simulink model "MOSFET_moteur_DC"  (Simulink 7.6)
settings: Solver=ode15s  StartTime=0.0  StopTime=0.1  RelTol=1e-3
InitFcn:
  | clc, close all
StopFcn:
  | close all, clc
  | load signaux_VitPos.mat
  | plotyy(x(1,:),x(2,:),x(1,:),x(3,:))
  | grid
  | title('Vitesse (rad/s) et Angle de rotation (rad)')
  | 
  | figure
  | load signaux_VI.mat
  | subplot 212
  | plot(y(1,:),y(2,:))
  | title('Courant de drain Id (A)')
  | grid
  | subplot 211
  | plot (y(1,:),y(3,:))
  | grid
  | title('Tension PWM de grille (V)')
libraries: fl_lib x14, nesl_utility x6, elec_lib x5

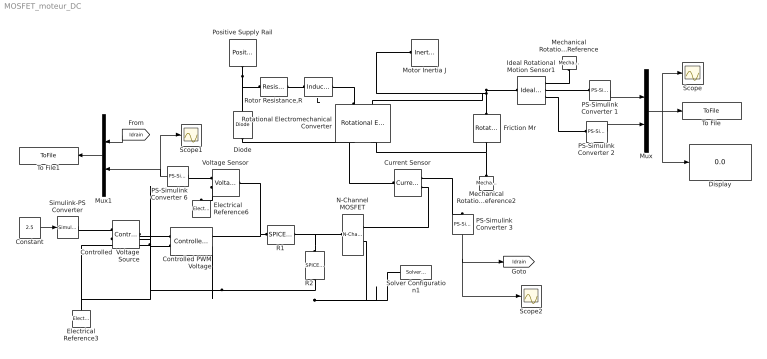
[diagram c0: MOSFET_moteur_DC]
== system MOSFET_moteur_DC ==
  Constant : Constant  Value=2.5
  Controlled  Voltage Source : fl_lib/Electrical/Electrical Sources/Controlled Voltage Source  DialogController=NetworkEngine.DynNeDlgSource  SystemSampleTime=-1  i_Log=off  v_Log=off  LocalVarNames=|i|v  LocalVarDescs=|i|v  LocalVarLogging=[0 0]
  Controlled PWM Voltage : elec_lib/Actuators & Drivers/Drivers/Controlled PWM Voltage  DialogController=NetworkEngine.DynNeDlgSource  SystemSampleTime=-1  F=1000 Hz  Vmin=0 V  Vmax=5 V  Vm=5 V  pwm_or_av=1  current_Log=off  voltage_Log=off  power_Log=off  LocalVarNames=|current|voltage|power  LocalVarDescs=|Load current (A)|Load voltage (V)|Load power (W)  LocalVarLogging=[0 0 0]
  Current Sensor : fl_lib/Electrical/Electrical Sensors/Current Sensor  DialogController=NetworkEngine.DynNeDlgSource  SystemSampleTime=-1  i1_Log=off  v1_Log=off  LocalVarNames=|i1|v1  LocalVarDescs=|i1|v1  LocalVarLogging=[0 0]
  Diode : fl_lib/Electrical/Electrical Elements/Diode  DialogController=NetworkEngine.DynNeDlgSource  SystemSampleTime=-1  Vf=0.6 V  Ron=0.3 Ohm  Goff=1e-08 1/Ohm  i_Log=off  v_Log=off  LocalVarNames=|i|v  LocalVarDescs=|i|v  LocalVarLogging=[0 0]
  Display : Display
  Electrical Reference3 : fl_lib/Electrical/Electrical Elements/Electrical Reference  DialogController=NetworkEngine.DynNeDlgSource  SystemSampleTime=-1  i_Log=off  LocalVarNames=|i  LocalVarDescs=|i  LocalVarLogging=[]
  Electrical Reference6 : fl_lib/Electrical/Electrical Elements/Electrical Reference  DialogController=NetworkEngine.DynNeDlgSource  SystemSampleTime=-1  i_Log=off  LocalVarNames=|i  LocalVarDescs=|i  LocalVarLogging=[]
  Friction Mr : fl_lib/Mechanical/Rotational Elements/Rotational Friction  DialogController=NetworkEngine.DynNeDlgSource  SystemSampleTime=-1  brkwy_trq=0.02e-3 N*m  Col_trq=0.02e-3 N*m  visc_coef=0 N*m/(rad/s)  trans_coef=10 s/rad  vel_thr=0.1 rad/s  t_Log=off  w_Log=off  LocalVarNames=|friction_torque|rel_velocity|power  LocalVarDescs=|Friction torque (N*m)|Relative velocity (rad/s)|Power (W)  LocalVarLogging=[0 0 0]
  Ideal Rotational Motion Sensor1 : fl_lib/Mechanical/Mechanical Sensors/Ideal Rotational Motion Sensor  DialogController=NetworkEngine.DynNeDlgSource  SystemSampleTime=-1  offset=0 rad  w_Log=off  t_Log=off  phi_Log=off  LocalVarNames=|w|t|phi  LocalVarDescs=|w|t|phi  LocalVarLogging=[]
  L : fl_lib/Electrical/Electrical Elements/Inductor  DialogController=NetworkEngine.DynNeDlgSource  SystemSampleTime=-1  l=12e-6 H  i0=0 A  r=0 Ohm  g=1e-09 1/Ohm  i_Log=off  v_Log=off  i_L_Log=off  LocalVarNames=|current|voltage|power  LocalVarDescs=|Inductor current (A) |Voltage across inductor (V)|Power (W)  LocalVarLogging=[0 0 0]
  Mechanical Rotational Reference : fl_lib/Mechanical/Rotational Elements/Mechanical Rotational Reference  DialogController=NetworkEngine.DynNeDlgSource  SystemSampleTime=-1  t_Log=off  LocalVarNames=|t  LocalVarDescs=|t  LocalVarLogging=[]
  Mechanical Rotational Reference2 : fl_lib/Mechanical/Rotational Elements/Mechanical Rotational Reference  DialogController=NetworkEngine.DynNeDlgSource  SystemSampleTime=-1  t_Log=off  LocalVarNames=|t  LocalVarDescs=|t  LocalVarLogging=[]
  Motor Inertia J : fl_lib/Mechanical/Rotational Elements/Inertia  DialogController=NetworkEngine.DynNeDlgSource  SystemSampleTime=-1  inertia=0.01 g*cm^2  initial_velocity=0 rad/s  t_Log=off  LocalVarNames=|torque|velocity  LocalVarDescs=|Inertia torque (N*m)|Inertia absolute velocity (rad/s)  LocalVarLogging=[0 0]
  Mux : Mux  Inputs=2
  Mux1 : Mux  Inputs=2
  N-Channel MOSFET : elec_lib/Semiconductor Devices/N-Channel MOSFET  DialogController=NetworkEngine.DynNeDlgSource  SystemSampleTime=-1  parameterization=1  Beta=5 A/V^2  Rds=0.025 Ohm  Id=6 A  Vgs=10 V  Vth=1.7 V  lam=0 1/V  RS=0.001 Ohm  RD=0.001 Ohm  C_param=1  C_GS=270 pF  C_GD=80 pF  C_iss=350 pF  C_rss=80 pF  LocalVarLogging=[]
  PS-Simulink Converter {1..3,6} (4 alike) : nesl_utility/PS-Simulink Converter  DialogController=NetworkEngine.DynNeUtilDlgSource  SystemSampleTime=-1  PhysicalDomain=network_engine_domain  LeftPortType=input  RightPortType=output  SubClassName=ps_output  Unit=1  AffineConversion=off
  Positive Supply Rail : elec_lib/Sources/Positive Supply Rail  DialogController=NetworkEngine.DynNeDlgSource  SystemSampleTime=-1  v0=15 V  current_Log=off  voltage_Log=off  power_Log=off  LocalVarNames=|current|voltage|power  LocalVarDescs=|Current (A)|Voltage (V)|Power (W)  LocalVarLogging=[0 0 0]
  R1 : elec_lib/Additional Components/SPICE-Compatible Components/Passive Devices/SPICE Resistor  DialogController=NetworkEngine.DynNeDlgSource  SystemSampleTime=-1  SCALE=1  R_param=1  R=1000 Ohm  RSH=0 Ohm  LENGTH=1e-06 m  WIDTH=1e-06 m  NARROW=0 m  T_param=1  TC1=0 1/K  TC2=0 1/K^2  TOFFSET=0 K  TFIXED=300.15 K  TMEAS=300.15 K  LocalVarLogging=[]
  R2 : elec_lib/Additional Components/SPICE-Compatible Components/Passive Devices/SPICE Resistor  DialogController=NetworkEngine.DynNeDlgSource  SystemSampleTime=-1  SCALE=1  R_param=1  R=100 kOhm  RSH=0 Ohm  LENGTH=1e-06 m  WIDTH=1e-06 m  NARROW=0 m  T_param=1  TC1=0 1/K  TC2=0 1/K^2  TOFFSET=0 K  TFIXED=300.15 K  TMEAS=300.15 K  LocalVarLogging=[]
  Rotational Electromechanical Converter : fl_lib/Electrical/Electrical Elements/Rotational Electromechanical Converter  DialogController=NetworkEngine.DynNeDlgSource  SystemSampleTime=-1  K=0.072e-3*60/(2*pi) s*V/rad  i_Log=off  v_Log=off  t_Log=off  w_Log=off  LocalVarNames=|current|voltage|power|torque|speed  LocalVarDescs=|Current (A)|Voltage (V)|Power (W)|Torque (Nm)|Angular speed (rad/s)  LocalVarLogging=[0 0 0 0 0]
  Rotor Resistance,R : fl_lib/Electrical/Electrical Elements/Resistor  Tag=Factory Generic  DialogController=NetworkEngine.DynNeDlgSource  SystemSampleTime=-1  R=3.9 Ohm  i_Log=off  v_Log=off  LocalVarNames=|current|voltage|power  LocalVarDescs=|Resistor current (A)|Voltage across resistor (V)|Power (W)  LocalVarLogging=[0 0 0]
  Scope : Scope
  Scope1 : Scope
  Scope2 : Scope
  Simulink-PS Converter : nesl_utility/Simulink-PS Converter  DialogController=NetworkEngine.DynNeUtilDlgSource  SystemSampleTime=-1  PhysicalDomain=network_engine_domain  LeftPortType=input  RightPortType=output  SubClassName=ps_input  Unit=1  AffineConversion=off  InputFilterTimeConstant=.001  UdotUserProvided=0
  Solver Configuration1 : nesl_utility/Solver Configuration  DialogController=NetworkEngine.DynNeUtilDlgSource  SystemSampleTime=-1  PhysicalDomain=network_engine_domain  LeftPortType=input  RightPortType=generic  SubClassName=solver  Accelerate=off  Profile=off  ResidualTolerance=1e-9  MaxNonlinIter=12  MaxModeIter=2  DoFixedCost=off  UseLocalSampling=off  DoDC=off  LinearAlgebra=Sparse  LocalSolverSampleTime=.001  LocalSolverChoice=NE_BACKWARD_EULER_ADVANCER  UseLocalSolver=off
  To File : ToFile  Filename=signaux_VitPos  MatrixName=x
  To File1 : ToFile  Filename=signaux_VI  MatrixName=y
  Voltage Sensor : fl_lib/Electrical/Electrical Sensors/Voltage Sensor  DialogController=NetworkEngine.DynNeDlgSource  SystemSampleTime=-1  i1_Log=off  v1_Log=off  LocalVarNames=|i1|v1  LocalVarDescs=|i1|v1  LocalVarLogging=[0 0]
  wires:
  Constant/1 -> Simulink-PS Converter/1
  PS-Simulink Converter 1/1 -> Mux/1
  PS-Simulink Converter 2/1 -> Mux/2
  Mux/1 -> To File/1, Scope/1, Display/1
  Mux1/1 -> To File1/1
  PS-Simulink Converter 6/1 -> Mux1/2, Scope1/1
  PS-Simulink Converter 3/1 -> [Idrain], Scope2/1
  [Idrain] -> Mux1/1
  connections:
  Positive Supply Rail/RConn1 -- Rotor Resistance,R/LConn1 -- Diode/RConn1
  Diode/LConn1 -- Rotational Electromechanical Converter/RConn1 -- Current Sensor/LConn1
  Friction Mr/RConn1 -- Rotational Electromechanical Converter/RConn2 -- Mechanical Rotational Reference2/LConn1
  L/LConn1 -- Rotor Resistance,R/RConn1
  Rotational Electromechanical Converter/LConn1 -- L/RConn1
  R2/LConn1 -- N-Channel MOSFET/LConn1 -- R1/LConn1
  Simulink-PS Converter/RConn1 -- Controlled  Voltage Source/RConn1
  Controlled  Voltage Source/LConn1 -- Controlled PWM Voltage/LConn1
  Mechanical Rotational Reference/LConn1 -- Ideal Rotational Motion Sensor1/RConn1
  Ideal Rotational Motion Sensor1/RConn2 -- PS-Simulink Converter 1/LConn1
  Ideal Rotational Motion Sensor1/RConn3 -- PS-Simulink Converter 2/LConn1
  R2/RConn1 -- Controlled PWM Voltage/RConn2 -- Electrical Reference3/LConn1 -- Controlled  Voltage Source/RConn2 -- Controlled PWM Voltage/LConn2 -- N-Channel MOSFET/RConn2 -- Solver Configuration1/RConn1
  Current Sensor/RConn2 -- N-Channel MOSFET/RConn1
  Current Sensor/RConn1 -- PS-Simulink Converter 3/LConn1
  Rotational Electromechanical Converter/LConn2 -- Motor Inertia J/LConn1 -- Ideal Rotational Motion Sensor1/LConn1 -- Friction Mr/LConn1
  R1/RConn1 -- Controlled PWM Voltage/RConn1 -- Voltage Sensor/LConn1
  Voltage Sensor/RConn2 -- Electrical Reference6/LConn1
  PS-Simulink Converter 6/LConn1 -- Voltage Sensor/RConn1
